ORGANIZATION_BLOCK OB 1
BEGIN
	CALL		FC 1
	CALL		FC 2
	CALL		FC 3
	CALL		FB 1, DB 2 (
		INPUT_VAR := 1
	)

//	U		"test_symbol_E"
//	=		"test_symbol_A"

END_ORGANIZATION_BLOCK



FUNCTION FC 1: VOID
BEGIN
	U		E 0.0
	=		A 0.0
END_FUNCTION



FUNCTION FC 2: VOID
TITLE = Shift register
BEGIN
	UN		T 10
	=		M 0.0
	L		S5T#200MS
	SV		T 10

	L		MD 4
	L		1
	==D
	S		M 0.1
	RRD		1
	==D
	R		M 0.1

	L		MD 4
	UD		L#-1
	L		1
	SPZ		_001
	TAK
	U		M 0.0
	SPBN		_001
	U		M 0.1
	SPBN		_000
	RLD		2
_000:	RRD		1
_001:	T		MD 4

	L		MD 4
	T		AD 4
	TAD
	T		AD 8
END_FUNCTION



FUNCTION FC 3: VOID
TITLE = DB usage example
BEGIN
	AUF		DB 1
	L		DBD 2
	T		MD 16
END_FUNCTION



FUNCTION_BLOCK FB 1
  VAR_INPUT
    INPUT_VAR : INT
  END_VAR
BEGIN
	NOP 0
END_FUNCTION_BLOCK



DATA_BLOCK DB 1
TITLE = This is global DB 1
STRUCT
	VAR1 : INT		// DBW0: VAR1 => 16 bit signed int
	VAR2 : DWORD	// DBD2: VAR2 => 32 bit unsigned dword
	VAR3 : WORD		// DBW6: VAR3 => 16 bit unsigned word
END_STRUCT
BEGIN
	VAR1 := 1337
	VAR2 := DW#16#DEADBEEF
	VAR3 := B#(1, 2)
END_DATA_BLOCK



DATA_BLOCK DB 2
TITLE = This is an instance DB for FB 1
FB 1
BEGIN
	INPUT_VAR := 123
END_DATA_BLOCK
